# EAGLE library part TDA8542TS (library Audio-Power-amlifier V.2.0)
2 ´ 0.7 W BTL audio amplifier
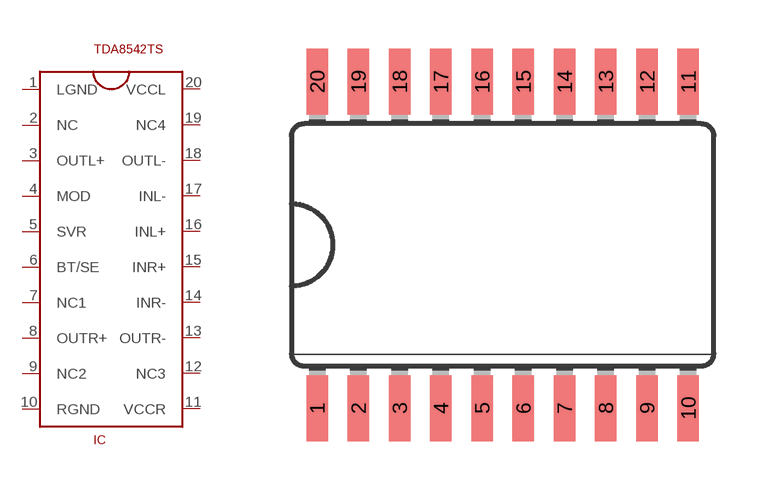
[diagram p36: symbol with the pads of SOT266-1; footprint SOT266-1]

Designator prefix IC

## TDA8542TS  [SOT266-1]
1  LGND  pwr
2  NC  nc
3  OUTL+  out
4  MOD
5  SVR
6  BT/SE
7  NC1  nc
8  OUTR+  out
9  NC2  nc
10  RGND  pwr
11  VCCR  pwr
12  NC3  nc
13  OUTR-  out
14  INR-  in
15  INR+  in
16  INL+  in
17  INL-  in
18  OUTL-  out
19  NC4  nc
20  VCCL  pwr

## Footprint SOT266-1 (pad centres in mm)
Small Outline Package
smd 0.66 x 2.032: 1 -5.715,-5.029; 2 -4.445,-5.029; 3 -3.175,-5.029; 4 -1.905,-5.029; 5 -0.635,-5.029; 6 0.635,-5.029; 7 1.905,-5.029; 8 3.175,-5.029; 9 4.445,-5.029; 10 5.715,-5.029; 11 5.715,5.029; 12 4.445,5.029; 13 3.175,5.029; 14 1.905,5.029; 15 0.635,5.029; 16 -0.635,5.029; 17 -1.905,5.029; 18 -3.175,5.029; 19 -4.445,5.029; 20 -5.715,5.029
